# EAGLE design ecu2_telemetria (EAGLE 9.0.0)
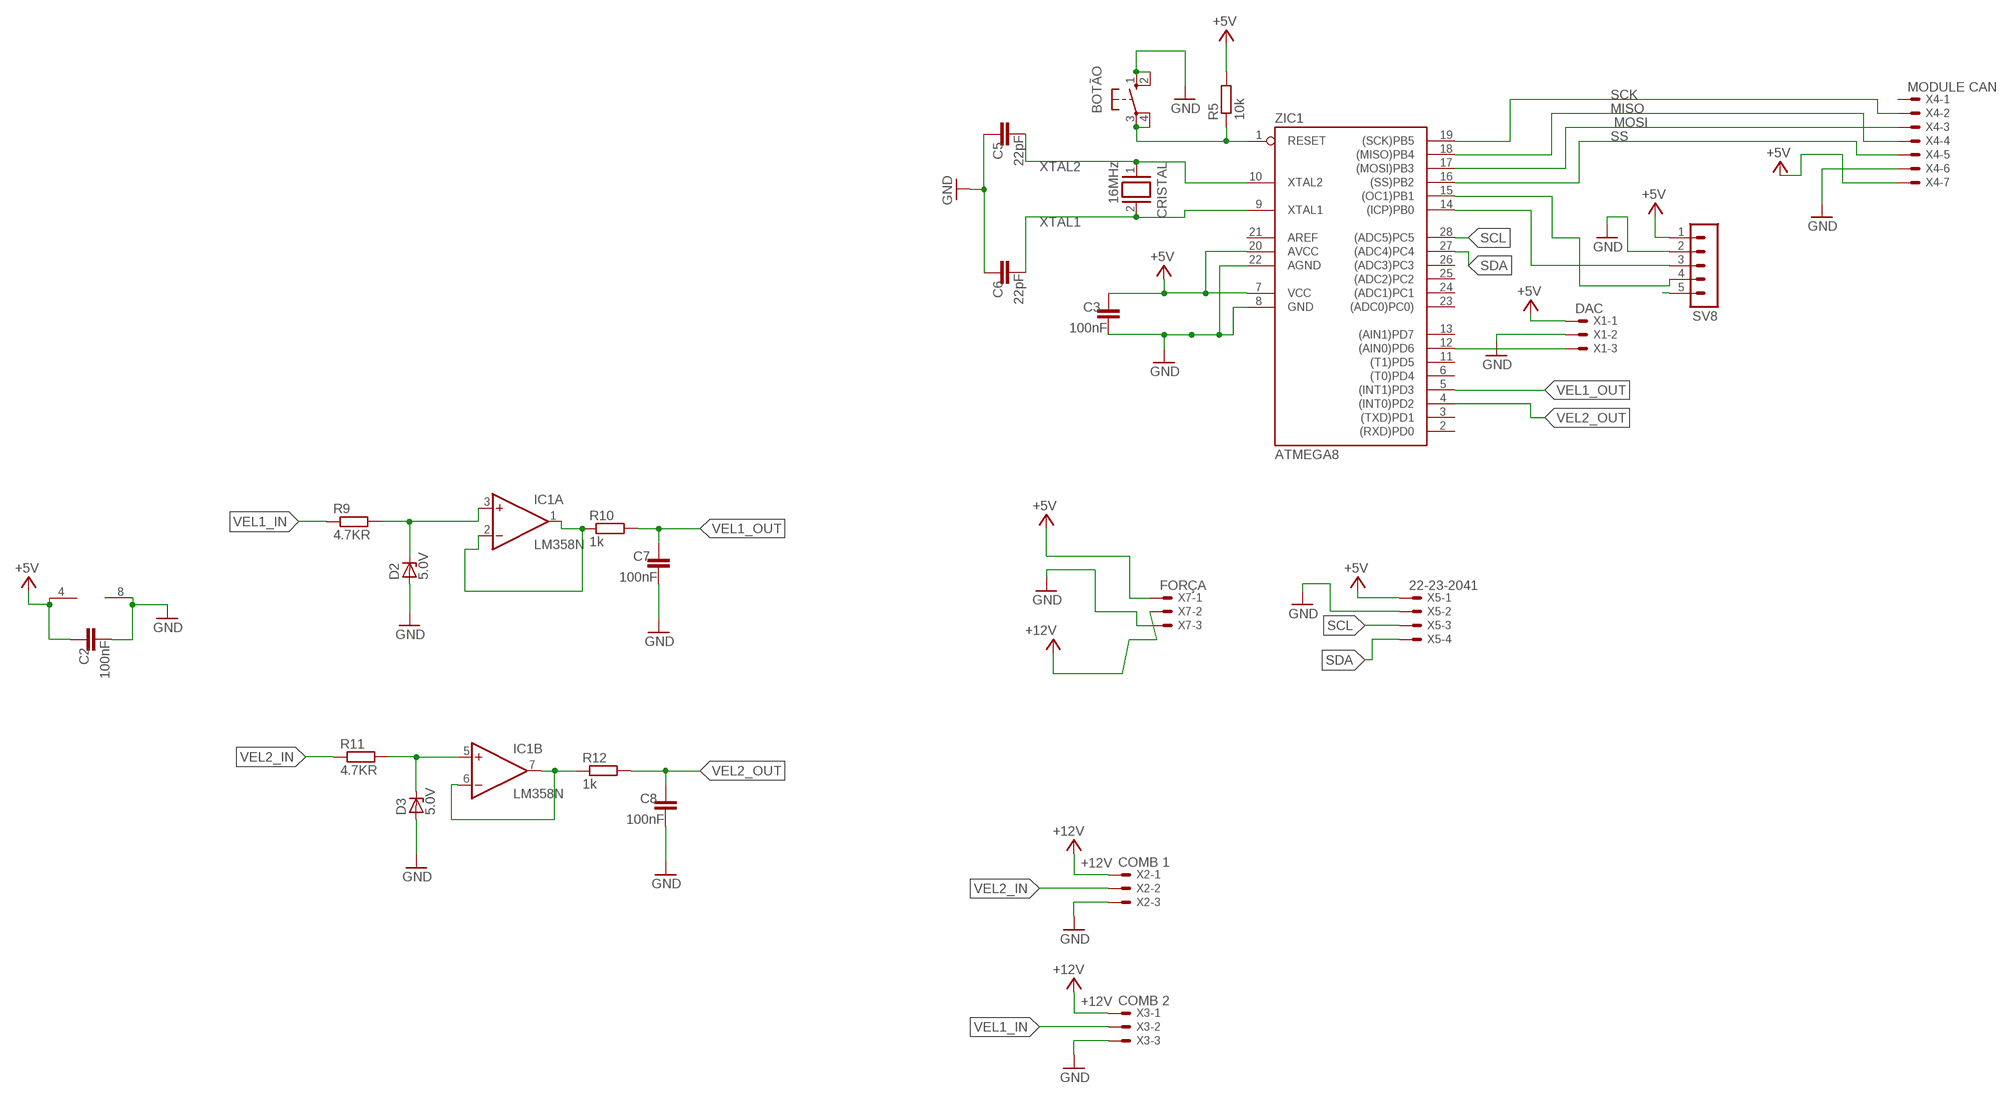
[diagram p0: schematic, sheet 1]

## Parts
BOTÃO  10-XX  [B3F-10XX]
C2  100nF  C5/2.5  [C5B2.5]
C3  100nF  C5/2.5  [C5B2.5]
C5  22pF  C5/2.5  [C5B2.5]
C6  22pF  C5/2.5  [C5B2.5]
C7  100nF  C5/2.5  [C5B2.5]
C8  100nF  C5/2.5  [C5B2.5]
CRISTAL  16MHz  XTAL/S  [QS]
D2  5.0V  ZENER-DIODEDO34-7  [DO34Z7]
D3  5.0V  ZENER-DIODEDO34-7  [DO34Z7]
IC1  LM358N  [DIL08]
R5  10k  R-EU_0207/7  [0207/7]
R9  4.7KR  R-EU_0207/7  [0207/7]
R10  1k  R-EU_0207/7  [0207/7]
R11  4.7KR  R-EU_0207/7  [0207/7]
R12  1k  R-EU_0207/7  [0207/7]
SV8  MA05-1  [MA05-1]
X1  DAC  22-23-2031  [22-23-2031]
X2  COMB 1  22-23-2031  [22-23-2031]
X3  COMB 2  22-23-2031  [22-23-2031]
X4  MODULE CAN  22-23-2071  [22-23-2071]
X5  22-23-2041  [22-23-2041]
X7  FORÇA  22-23-2031  [22-23-2031]
ZIC1  ATMEGA8  AT90S4433P  [DIL28-3]

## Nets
+5V: C2.2 C3.2 IC1.4(P:V-) R5.2 SV8.1 X1.1 X4.7 X5.1 X7.1 ZIC1.7(VCC) ZIC1.20(AVCC)
+12V: X2.1 X3.1 X7.2
GND: BOTÃO.1(S) BOTÃO.2(S1) C2.1 C3.1 C5.2 C6.2 C7.1 C8.1 D2.A D3.A IC1.8(P:V+) SV8.2 X1.2 X2.3 X3.3 X4.6 X5.2 X7.3 ZIC1.8(GND) ZIC1.22(AGND)
IO8: SV8.3 ZIC1.14((ICP)PB0)
IO9: SV8.4 ZIC1.15((OC1)PB1)
MISO: X4.4 ZIC1.18((MISO)PB4)
MOSI: X4.3 ZIC1.17((MOSI)PB3)
N$3: X1.3 ZIC1.12((AIN0)PD6)
N$5: D2.C IC1.3(A:+IN) R9.2
N$6: SV8.5
N$9: BOTÃO.3(P) BOTÃO.4(P1) R5.1 ZIC1.1(RESET)
N$12: IC1.1(A:OUT) IC1.2(A:-IN) R10.1
N$13: D3.C IC1.5(B:+IN) R11.2
N$14: IC1.6(B:-IN) IC1.7(B:OUT) R12.1
SCK: X4.2 ZIC1.19((SCK)PB5)
SCL: X5.3 ZIC1.28((ADC5)PC5)
SDA: X5.4 ZIC1.27((ADC4)PC4)
SS: X4.5 ZIC1.16((SS)PB2)
VEL1_IN: R9.1 X3.2
VEL1_OUT: C7.2 R10.2 ZIC1.5((INT1)PD3)
VEL2_IN: R11.1 X2.2
VEL2_OUT: C8.2 R12.2 ZIC1.4((INT0)PD2)
XTAL1: C6.1 CRISTAL.2 ZIC1.9(XTAL1)
XTAL2: C5.1 CRISTAL.1 ZIC1.10(XTAL2)
Unconnected: X4.1 ZIC1.2((RXD)PD0) ZIC1.3((TXD)PD1) ZIC1.6((T0)PD4) ZIC1.11((T1)PD5) ZIC1.13((AIN1)PD7) ZIC1.21(AREF) ZIC1.23((ADC0)PC0)) ZIC1.24((ADC1)PC1) ZIC1.25((ADC2)PC2) ZIC1.26((ADC3)PC3)

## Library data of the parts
BOTÃO = switch-omron:10-XX: OMRON SWITCH; MPN: B3F-1000; OC_FARNELL: 176432; OC_NEWARK: 36M3542
C2 C3 C5-C8 = capacitor-wima:C: CAPACITOR
CRISTAL = special:XTAL/S: CRYSTAL
D2 D3 = diode:ZENER-DIODE: Z-Diode
IC1 = linear:LM358: OP AMP also LM158; LM258; LM2904 Source: http://cache.national.com/ds/LM/LM158.pdf
R5 R9-R12 = resistor:R-EU_: RESISTOR, European symbol
SV8 = con-lstb:MA05-1: PIN HEADER; OC_FARNELL: unknown; OC_NEWARK: unknown
X1-X3 X7 = con-molex:22-23-2031: .100" (2.54mm) Center Header - 3 Pin; MF: MOLEX; MPN: 22-23-2031; OC_FARNELL: 1462950; OC_NEWARK: 30C0862
X4 = con-molex:22-23-2071: .100" (2.54mm) Center Header - 7 Pin; MF: MOLEX; MPN: 22-23-2071; OC_FARNELL: 1654534; OC_NEWARK: 56H0445
X5 = con-molex:22-23-2041: .100" (2.54mm) Center Header - 4 Pin; MF: MOLEX; MPN: 22-23-2041; OC_FARNELL: 1462920; OC_NEWARK: 38C0355
ZIC1 = atmel:AT90S4433: MICROCONTROLLER 4 Kbytes FLASH 128 bytes SRAM 256 bytes EEPROM UART 6-channel 10 bit ADC

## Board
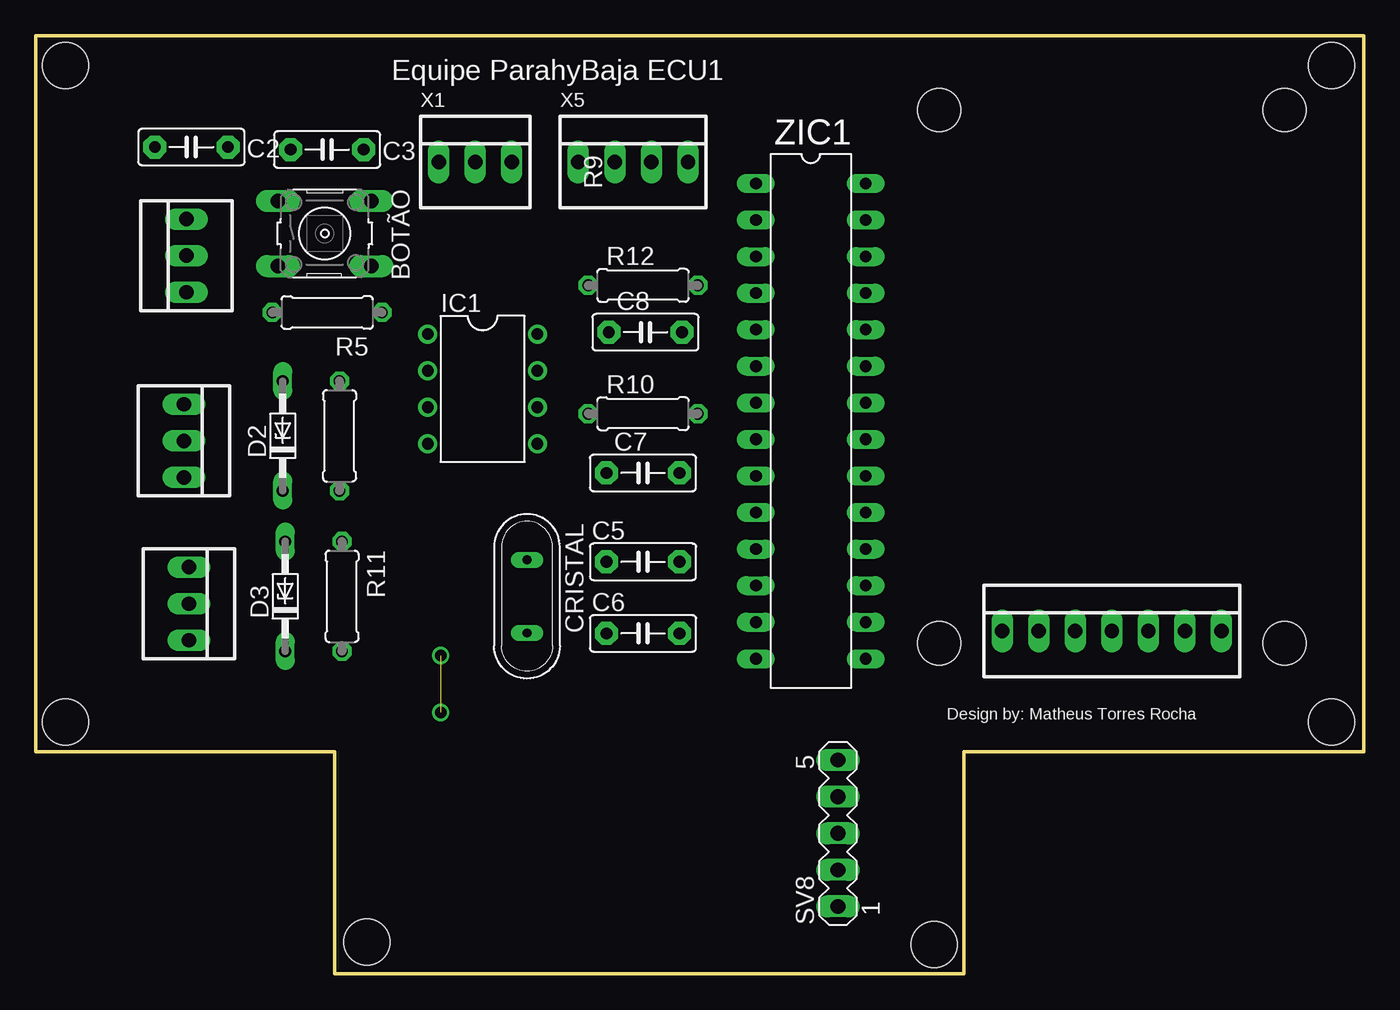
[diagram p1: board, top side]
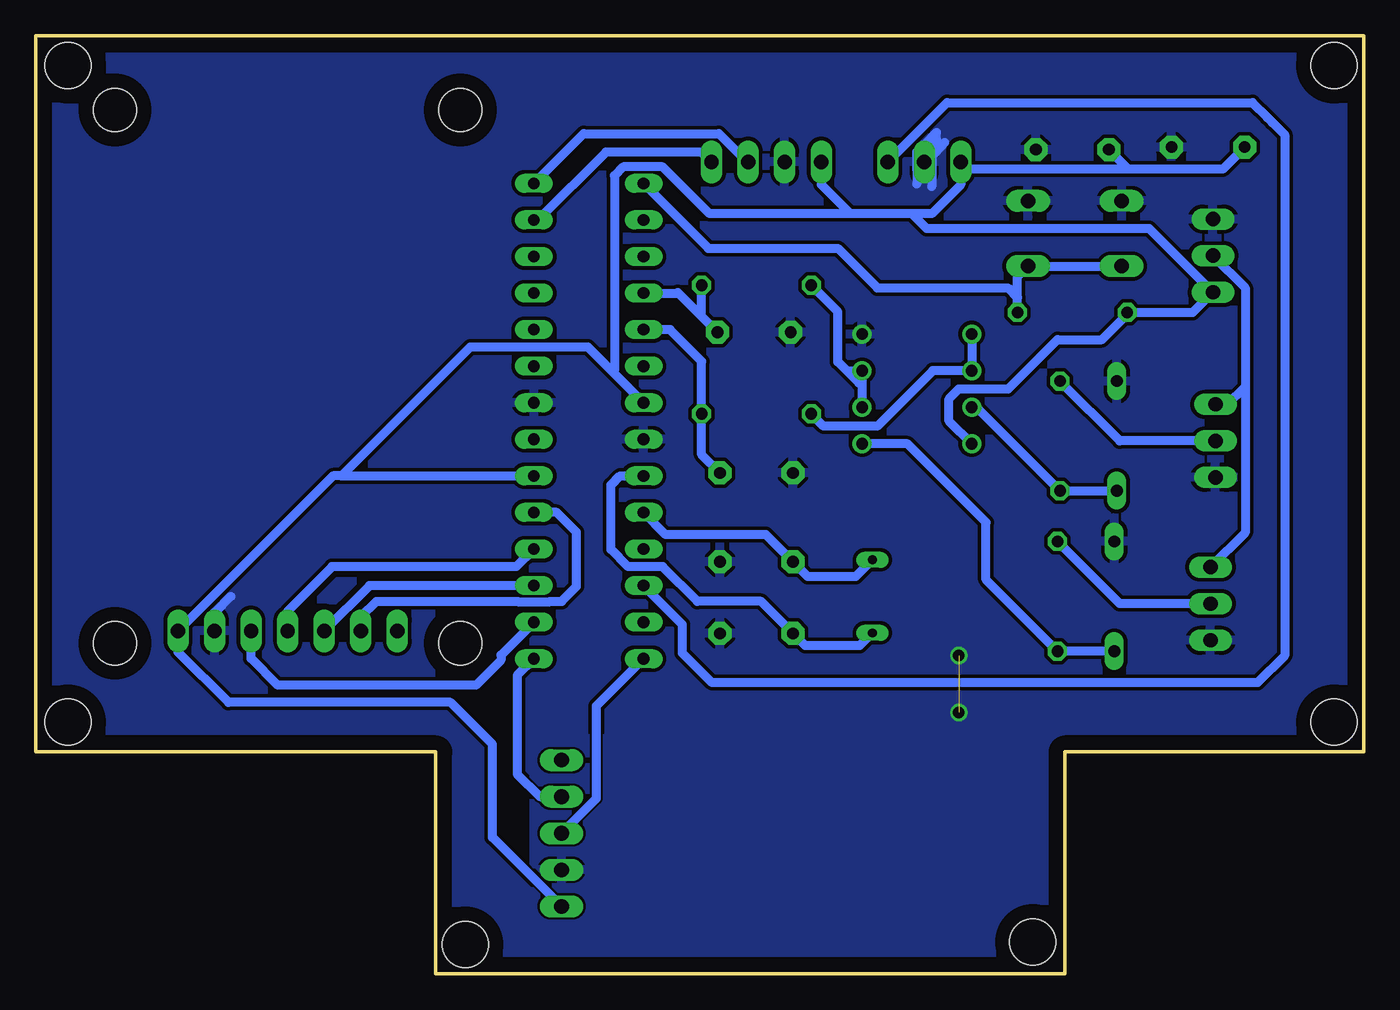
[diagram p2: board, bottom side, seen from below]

Size 92.24 x 65.15 mm. Coordinates in mm from the lower left corner, seen from the top.
Outline: 0,65.15 0,15.43 20.75,15.43 20.75,0 64.47,0 64.47,15.43 92.24,15.43 92.24,65.15 0,65.15
Copper layers (1*16): Top 0.035mm / dielectric 1.5mm / Bottom 0.035mm
Design rules "default": minimum track width 6mil, minimum drill 0.35mm, track to track 6mil, track to pad 6mil, pad to pad 6mil, via to via 6mil, smd to smd 6mil, copper to edge 40mil, drill to drill 6mil, minimum pad ring 10mil, minimum via ring 8mil, stop-mask expansion 4mil, vias tented up to drill 0mil, thermal gap 10mil
Holes 3 mm at 62.75,60.01 86.75,60.01 62.75,22.97 86.75,22.97
Holes 3.2 mm at 2.06,63.09 2.06,17.49 22.97,2.23 62.41,2.06 90.01,17.49 90.01,63.09

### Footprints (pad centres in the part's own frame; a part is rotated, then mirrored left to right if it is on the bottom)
B3F-10XX = drill 1.016 long: 1 -3.251,2.261; 2 3.251,2.261; 3 -3.251,-2.261; 4 3.251,-2.261
C5B2.5 = drill 0.813 pad 1.6 octagon: 1 -2.54,0; 2 2.54,0
QS = drill 0.61 long: 1 -2.54,0; 2 2.54,0
DO34Z7 = drill 0.813 long: A 3.81,0; C -3.81,0
DIL08 = drill 0.813 pad 1.27: 1 -3.81,-3.81; 2 -1.27,-3.81; 3 1.27,-3.81; 4 3.81,-3.81; 5 3.81,3.81; 6 1.27,3.81; 7 -1.27,3.81; 8 -3.81,3.81
0207/7 = drill 0.813 octagon: 1 -3.81,0; 2 3.81,0
MA05-1 = drill 1.016 long: 1 -5.08,0; 2 -2.54,0; 3 0,0; 4 2.54,0; 5 5.08,0
22-23-2031 = drill 1 long: 1 -2.54,0; 2 0,0; 3 2.54,0
22-23-2071 = drill 1 long: 1 -7.62,0; 2 -5.08,0; 3 -2.54,0; 4 0,0; 5 2.54,0; 6 5.08,0; 7 7.62,0
22-23-2041 = drill 1 long: 1 -3.81,0; 2 -1.27,0; 3 1.27,0; 4 3.81,0
DIL28-3 = drill 0.813 long: 1 -16.51,-3.81; 2 -13.97,-3.81; 3 -11.43,-3.81; 4 -8.89,-3.81; 5 -6.35,-3.81; 6 -3.81,-3.81; 7 -1.27,-3.81; 8 1.27,-3.81; 9 3.81,-3.81; 10 6.35,-3.81; 11 8.89,-3.81; 12 11.43,-3.81; 13 13.97,-3.81; 14 16.51,-3.81; 15 16.51,3.81; 16 13.97,3.81; 17 11.43,3.81; 18 8.89,3.81; 19 6.35,3.81; 20 3.81,3.81; 21 1.27,3.81; 22 -1.27,3.81; 23 -3.81,3.81; 24 -6.35,3.81; 25 -8.89,3.81; 26 -11.43,3.81; 27 -13.97,3.81; 28 -16.51,3.81

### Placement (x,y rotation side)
BOTÃO  20.06,51.43 0 top
C2  10.8,57.44 180 top
C3  20.23,57.26 180 top
C5  42.18,28.63 0 top
C6  42.18,23.66 0 top
C7  42.18,34.8 0 top
C8  42.35,44.58 0 top
CRISTAL  34.12,26.23 270 top
D2  17.14,37.38 90 top
D3  17.32,26.23 90 top
IC1  31.03,40.63 270 top
R5  20.23,45.95 180 top
R9  21.09,37.38 270 top
R10  42.18,38.92 0 top
R11  21.26,26.23 270 top
R12  42.18,47.83 0 top
SV8  55.72,9.77 90 top
X1  30.52,56.41 0 top
X2  10.63,25.72 270 top
X3  10.29,37.03 270 top
X4  74.75,23.83 0 top
X5  41.49,56.41 0 top
X7  10.46,49.89 90 top
ZIC1  53.84,38.41 270 top

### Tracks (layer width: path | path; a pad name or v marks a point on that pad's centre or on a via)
+5V
  Bottom 0.61: 58.16,34.6 ZIC1.20 71.02,34.6 | SV8.1 60.52,9.49 60.52,15.95 63.44,18.86 78.87,18.86 82.37,22.36 X4.7 71.61,34.6 71.02,34.6 | IC1.4 28.8,38.41 28.8,39.95 28.12,40.63 24.69,40.63 21.26,44.06 18.17,44.06 16.42,45.82 R5.2 11.86,45.95 X7.1 14.88,51.78 30.35,51.78 31.38,52.81 | C2.2 9.79,55.91 16.34,55.91 | 16.34,55.91 C3.2 | 16.34,55.91 27.48,55.91 X1.1 27.98,54.83 30,52.81 31.38,52.81 | 31.38,52.81 35.66,52.81 | 35.66,52.81 45.43,52.81 48.69,56.06 51.44,56.06 52.05,55.45 52.05,41.9 52.15,41.8 | X5.1 37.68,54.83 35.66,52.81 | ZIC1.7 52.15,41.8 | 52.15,41.8 53.9,43.55 62.06,43.55 71.02,34.6
+12V
  Bottom 0.61: X7.2 8.23,47.66 8.23,40.81 | 8.23,40.81 9.46,39.57 X3.1 | 8.23,40.81 8.23,30.66 X2.1
GND  (via drill 0.8)  (1 unrouted)
  Bottom 0.61: 78.7,26.23 79.83,25.1 X4.6 | 30.52,57.61 29.66,58.46 29.66,57.95 30.52,57.09 X1.2 | X1.2 29.32,57.61 29.24,57.61 | 29.24,57.61 29.11,57.74 | 29.24,57.61 30,56.85 | 30,56.85 30,54.69 | 30,56.85 30,57.09 30.52,57.61 | X1.2 31.03,55.89 | 31.03,55.89 31.03,54.86 | 31.03,55.89 31.03,57.09 30.52,57.61
  other vias: 28.12,22.12 28.12,18.17
  pour Bottom (isolate 0.254): 1.54,65.15 92.24,65.15 92.24,15.6 92.24,15.43 64.47,15.43 64.47,0 20.75,0 20.75,15.43 0,15.43 0,65.15 1.37,65.15
IO8
  Bottom 0.61: ZIC1.14 53.32,18.6 53.32,12.17 SV8.3
IO9
  Bottom 0.61: ZIC1.15 58.81,20.73 58.81,13.89 57.23,12.31 SV8.4
MISO
  Bottom 0.61: ZIC1.18 58.87,28.29 71.67,28.29 74.75,25.2 X4.4
MODULE_CAN
  pour Bottom (isolate 0.406): 60.86,21.09 88.64,21.09 88.64,61.89 60.86,61.89
MOSI
  Bottom 0.61: ZIC1.17 69.07,26.98 X4.3
N$1
  pour Bottom: 57.78,2.74 26.92,2.74 26.92,16.46 57.78,16.46
N$3
  Bottom 0.61: ZIC1.12 47.32,24.27 47.32,22.29 45.26,20.23 7.37,20.23 5.49,22.12 5.49,58.29 6.34,59.15 6.69,59.49 7.72,60.52 28.94,60.52 X1.3
N$5
  Bottom 0.61: D2.C R9.2 26.89,39.36 IC1.3
N$9
  Bottom 0.61: R5.1 24.04,46.98 | 24.04,46.98 24.04,48.44 BOTÃO.4 BOTÃO.3 | ZIC1.1 45.52,50.41 36.52,50.41 33.78,47.66 24.73,47.66 24.04,46.98
N$12
  Bottom 0.61: IC1.1 IC1.2 29.93,41.9 33.78,38.06 37.51,38.06 R10.1
N$13
  Bottom 0.61: IC1.5 31.68,36.82 26.23,31.38 26.23,27.39 R11.2 D3.C
N$14
  Bottom 0.61: 35.9,41.9 36.52,42.52 36.52,45.99 R12.1 | 35.9,41.9 IC1.7 | 35.9,41.9 35.06,41.06 | 35.06,41.06 34.84,40.84 | 34.84,40.84 IC1.6 | IC1.7 35.06,41.69 35.06,41.06 | IC1.7 34.84,40.84
SCK
  Bottom 0.61: X4.2 69.67,24.8 68.58,25.89 58.8,25.89 58.77,25.86 56.52,25.86 56.49,25.89 55.72,25.89 54.69,26.92 54.69,30.69 56.06,32.06 ZIC1.19
SCL
  Bottom 0.61: X5.3 42.83,56.41 44.8,58.37 54.19,58.37 ZIC1.28
SDA
  Bottom 0.61: X5.4 45.99,57.09 52.64,57.09 57.35,52.38 ZIC1.27
SS
  Bottom 0.61: ZIC1.16 59.93,22.15 59.93,21.81 61.68,20.06 75.44,20.06 77.29,21.91 X4.5
VEL1_IN
  Bottom 0.61: X3.2 16.94,37.03 R9.1
VEL1_OUT
  Bottom 0.61: C7.2 45.99,36.08 R10.2 45.99,42.56 48.18,44.76 ZIC1.5
VEL2_IN
  Bottom 0.61: X2.2 16.94,25.72 R11.1
VEL2_OUT
  Bottom 0.61: C8.2 45.99,45.68 | 45.99,45.68 R12.2 | ZIC1.4 47.69,47.3 47.66,47.32 47.63,47.32 45.99,45.68
XTAL1
  Bottom 0.61: ZIC1.9 51.64,34.6 52.29,33.95 52.29,29.49 51.09,28.29 48.69,28.29 46.29,25.89 41.87,25.89 39.88,23.9 C6.1 38.78,22.8 35.01,22.8 CRISTAL.2
XTAL2
  Bottom 0.61: ZIC1.10 48.49,30.52 41.52,30.52 C5.1 38.61,27.6 35.29,27.6 CRISTAL.1

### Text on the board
tNames: Equipe ParahyBaja ECU1 | Design by: Matheus Torres Rocha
